(* Logix 5000 AddOnInstructionDefinition export Banner_R90C_R95C_PD_v4; software revision 33.00 *)

TYPE Banner_R90C_R95C_PDI_Discrete_v4 :
STRUCT
   P1_Input_1 : SINT;   // 0 = Inactive, 1 = Active. Port 1 Discrete 1 Input State.
   P1_Input_2 : SINT;   // 0 = Inactive, 1 = Active. Port 1 Discrete 2 Input State.
   P2_Input_1 : SINT;   // 0 = Inactive, 1 = Active. Port 1 Discrete 1 Input State.
   P2_Input_2 : SINT;   // 0 = Inactive, 1 = Active. Port 1 Discrete 2 Input State.
   P3_Input_1 : SINT;   // 0 = Inactive, 1 = Active. Port 1 Discrete 1 Input State.
   P3_Input_2 : SINT;   // 0 = Inactive, 1 = Active. Port 1 Discrete 2 Input State.
   P4_Input_1 : SINT;   // 0 = Inactive, 1 = Active. Port 1 Discrete 1 Input State.
   P4_Input_2 : SINT;   // 0 = Inactive, 1 = Active. Port 1 Discrete 2 Input State.
   P5_Input_1 : SINT;   // 0 = Inactive, 1 = Active. Port 1 Discrete 1 Input State.
   P5_Input_2 : SINT;   // 0 = Inactive, 1 = Active. Port 1 Discrete 2 Input State.
   P6_Input_1 : SINT;   // 0 = Inactive, 1 = Active. Port 1 Discrete 1 Input State.
   P6_Input_2 : SINT;   // 0 = Inactive, 1 = Active. Port 1 Discrete 2 Input State.
   P7_Input_1 : SINT;   // 0 = Inactive, 1 = Active. Port 1 Discrete 1 Input State.
   P7_Input_2 : SINT;   // 0 = Inactive, 1 = Active. Port 1 Discrete 2 Input State.
   P8_Input_1 : SINT;   // 0 = Inactive, 1 = Active. Port 1 Discrete 1 Input State.
   P8_Input_2 : SINT;   // 0 = Inactive, 1 = Active. Port 1 Discrete 2 Input State.
END_STRUCT
END_TYPE

TYPE Banner_R90C_R95C_PDI_v4 :   // UDT with all of the variables needed to control an R90C-4B21-KQ or R95C-8B21-KQ.
STRUCT
   Discrete_Info : Banner_R90C_R95C_PDI_Discrete_v4;
   Measurement_1 : DINT;
   Measurement_2 : DINT;
   Measurement_3 : DINT;
   Measurement_4 : DINT;
END_STRUCT
END_TYPE

TYPE Banner_R90C_R95C_PDIO_v4 :   // UDT with all of the variables needed to control an R90C-4B21-KQ or R95C-8B21-KQ.
STRUCT
   PDI : Banner_R90C_R95C_PDI_v4;
   PDO : Banner_R90C_R95C_PDO_v4;
   DTI : SINT[18];
   DTO : SINT[2];
END_STRUCT
END_TYPE

TYPE Banner_R90C_R95C_PDO_v4 :   // UDT with all of the variables needed to control an R90C-4B21-KQ or R95C-8B21-KQ.
STRUCT
   P1_Output_2 : SINT;   // 0 = Off, 1 = On
   P2_Output_2 : SINT;   // 0 = Off, 1 = On
   P3_Output_2 : SINT;   // 0 = Off, 1 = On
   P4_Output_2 : SINT;   // 0 = Off, 1 = On
   P5_Output_2 : SINT;   // 0 = Off, 1 = On
   P6_Output_2 : SINT;   // 0 = Off, 1 = On
   P7_Output_2 : SINT;   // 0 = Off, 1 = On
   P8_Output_2 : SINT;   // 0 = Off, 1 = On
END_STRUCT
END_TYPE

ADD_ON_INSTRUCTION Banner_R90C_R95C_PD_v4   (* revision 4.0, vendor Banner Engineering *)
// AOI that used with the R90C-4B21-KQ and he R95C-8B21-KQ Hub.
VAR_IN_OUT
   PD : Banner_R90C_R95C_PDIO_v4; {required}
END_VAR
VAR_INPUT
   Type : SINT; {required}
   Byte_Swap : BOOL; {required}
END_VAR
VAR
   TempOut : SINT[2]; {access None}
   TempIn : SINT[18]; {access None}
END_VAR

ROUTINE Logic   (* ladder *)
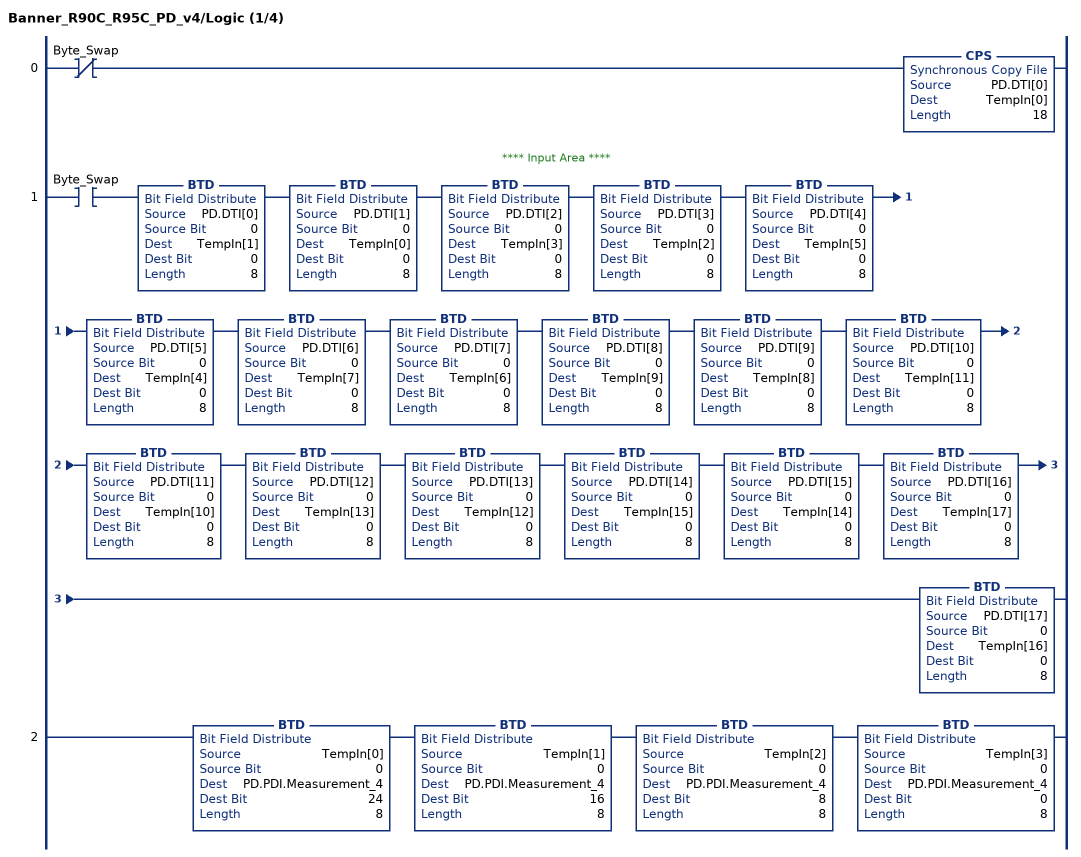
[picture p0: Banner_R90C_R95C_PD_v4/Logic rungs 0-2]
   0: XIO(Byte_Swap)CPS(PD.DTI[0],TempIn[0],18);
   // **** Input Area ****
   1: XIC(Byte_Swap)BTD(PD.DTI[0],0,TempIn[1],0,8)BTD(PD.DTI[1],0,TempIn[0],0,8)BTD(PD.DTI[2],0,TempIn[3],0,8)BTD(PD.DTI[3],0,TempIn[2],0,8)BTD(PD.DTI[4],0,TempIn[5],0,8)BTD(PD.DTI[5],0,TempIn[4],0,8)BTD(PD.DTI[6],0,TempIn[7],0,8)BTD(PD.DTI[7],0,TempIn[6],0,8)BTD(PD.DTI[8],0,TempIn[9],0,8)BTD(PD.DTI[9],0,TempIn[8],0,8)BTD(PD.DTI[10],0,TempIn[11],0,8)BTD(PD.DTI[11],0,TempIn[10],0,8)BTD(PD.DTI[12],0,TempIn[13],0,8)BTD(PD.DTI[13],0,TempIn[12],0,8)BTD(PD.DTI[14],0,TempIn[15],0,8)BTD(PD.DTI[15],0,TempIn[14],0,8)BTD(PD.DTI[16],0,TempIn[17],0,8)BTD(PD.DTI[17],0,TempIn[16],0,8);
   2: BTD(TempIn[0],0,PD.PDI.Measurement_4,24,8)BTD(TempIn[1],0,PD.PDI.Measurement_4,16,8)BTD(TempIn[2],0,PD.PDI.Measurement_4,8,8)BTD(TempIn[3],0,PD.PDI.Measurement_4,0,8);
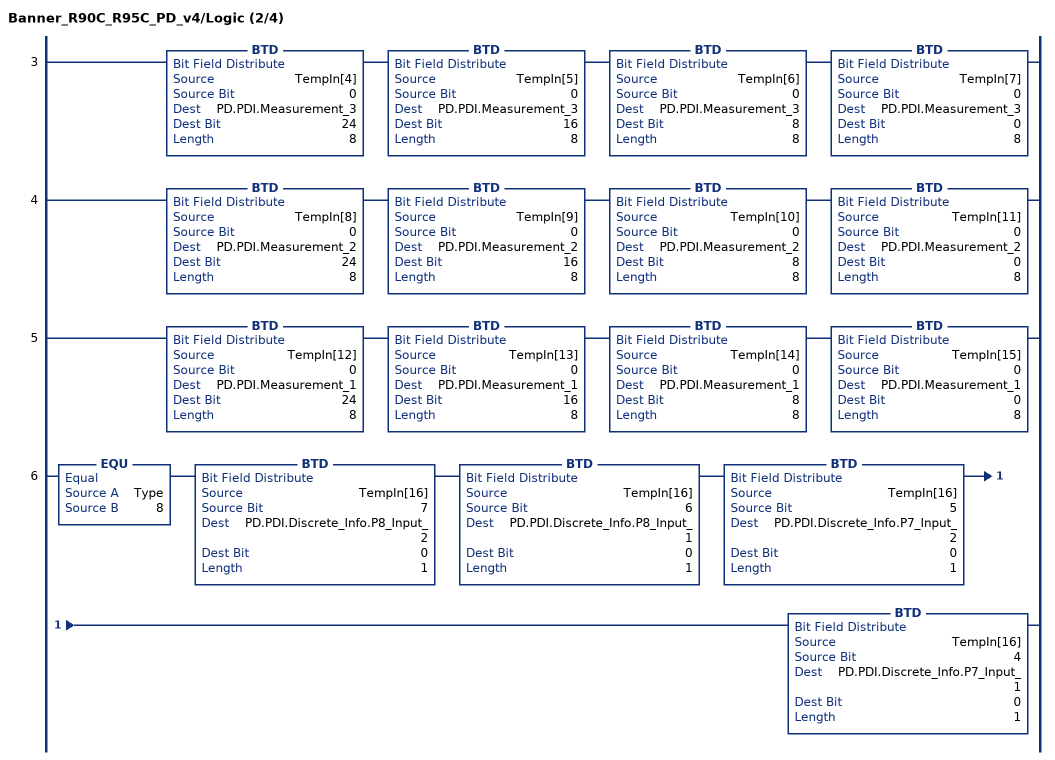
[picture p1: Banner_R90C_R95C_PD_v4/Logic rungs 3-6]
   3: BTD(TempIn[4],0,PD.PDI.Measurement_3,24,8)BTD(TempIn[5],0,PD.PDI.Measurement_3,16,8)BTD(TempIn[6],0,PD.PDI.Measurement_3,8,8)BTD(TempIn[7],0,PD.PDI.Measurement_3,0,8);
   4: BTD(TempIn[8],0,PD.PDI.Measurement_2,24,8)BTD(TempIn[9],0,PD.PDI.Measurement_2,16,8)BTD(TempIn[10],0,PD.PDI.Measurement_2,8,8)BTD(TempIn[11],0,PD.PDI.Measurement_2,0,8);
   5: BTD(TempIn[12],0,PD.PDI.Measurement_1,24,8)BTD(TempIn[13],0,PD.PDI.Measurement_1,16,8)BTD(TempIn[14],0,PD.PDI.Measurement_1,8,8)BTD(TempIn[15],0,PD.PDI.Measurement_1,0,8);
   6: EQU(Type,8)BTD(TempIn[16],7,PD.PDI.Discrete_Info.P8_Input_2,0,1)BTD(TempIn[16],6,PD.PDI.Discrete_Info.P8_Input_1,0,1)BTD(TempIn[16],5,PD.PDI.Discrete_Info.P7_Input_2,0,1)BTD(TempIn[16],4,PD.PDI.Discrete_Info.P7_Input_1,0,1);
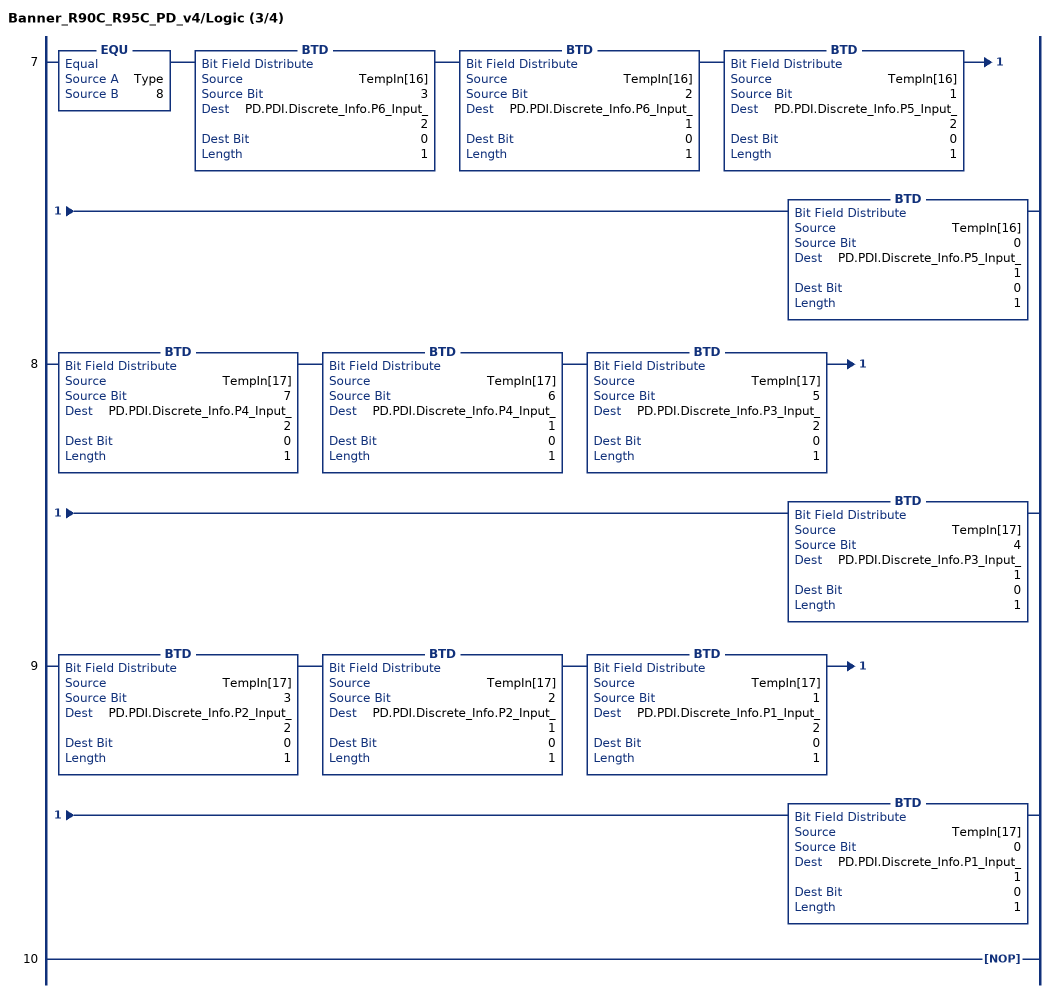
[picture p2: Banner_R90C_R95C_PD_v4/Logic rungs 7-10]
   7: EQU(Type,8)BTD(TempIn[16],3,PD.PDI.Discrete_Info.P6_Input_2,0,1)BTD(TempIn[16],2,PD.PDI.Discrete_Info.P6_Input_1,0,1)BTD(TempIn[16],1,PD.PDI.Discrete_Info.P5_Input_2,0,1)BTD(TempIn[16],0,PD.PDI.Discrete_Info.P5_Input_1,0,1);
   8: BTD(TempIn[17],7,PD.PDI.Discrete_Info.P4_Input_2,0,1)BTD(TempIn[17],6,PD.PDI.Discrete_Info.P4_Input_1,0,1)BTD(TempIn[17],5,PD.PDI.Discrete_Info.P3_Input_2,0,1)BTD(TempIn[17],4,PD.PDI.Discrete_Info.P3_Input_1,0,1);
   9: BTD(TempIn[17],3,PD.PDI.Discrete_Info.P2_Input_2,0,1)BTD(TempIn[17],2,PD.PDI.Discrete_Info.P2_Input_1,0,1)BTD(TempIn[17],1,PD.PDI.Discrete_Info.P1_Input_2,0,1)BTD(TempIn[17],0,PD.PDI.Discrete_Info.P1_Input_1,0,1);
   10: NOP();
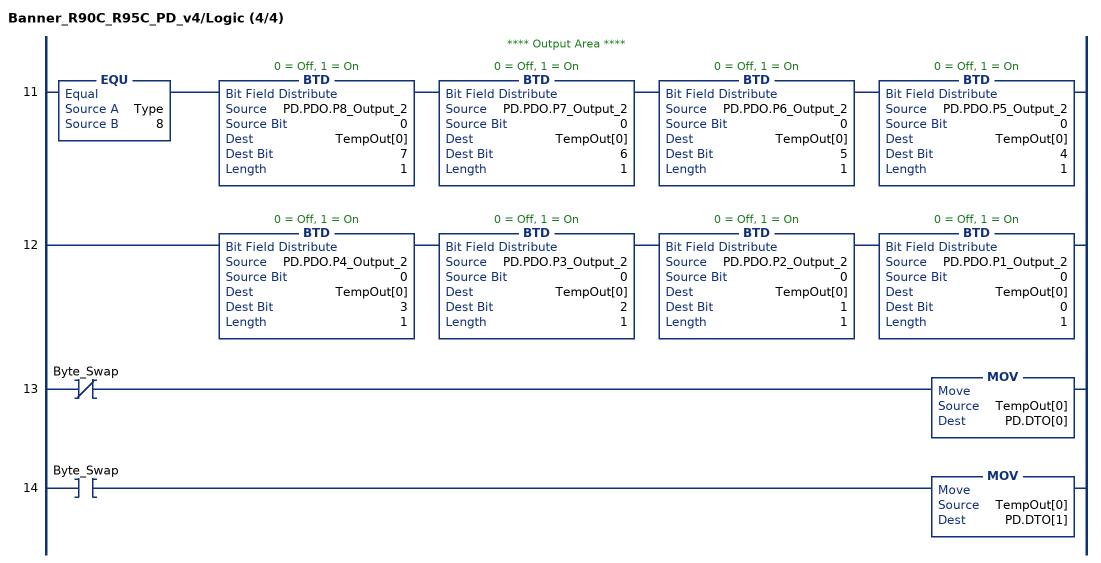
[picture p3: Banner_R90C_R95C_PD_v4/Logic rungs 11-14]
   // **** Output Area ****
   11: EQU(Type,8)BTD(PD.PDO.P8_Output_2,0,TempOut[0],7,1)BTD(PD.PDO.P7_Output_2,0,TempOut[0],6,1)BTD(PD.PDO.P6_Output_2,0,TempOut[0],5,1)BTD(PD.PDO.P5_Output_2,0,TempOut[0],4,1);
   12: BTD(PD.PDO.P4_Output_2,0,TempOut[0],3,1)BTD(PD.PDO.P3_Output_2,0,TempOut[0],2,1)BTD(PD.PDO.P2_Output_2,0,TempOut[0],1,1)BTD(PD.PDO.P1_Output_2,0,TempOut[0],0,1);
   13: XIO(Byte_Swap)MOV(TempOut[0],PD.DTO[0]);
   14: XIC(Byte_Swap)MOV(TempOut[0],PD.DTO[1]);
END_ROUTINE
END_ADD_ON_INSTRUCTION
